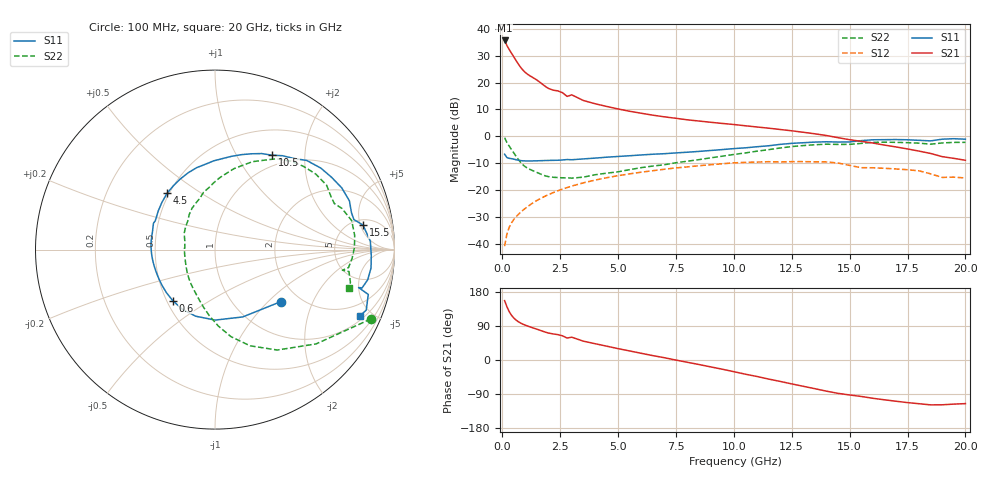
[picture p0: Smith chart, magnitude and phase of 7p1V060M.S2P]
! Infineon Technologies  Discrete & RF Semiconductors
! bfp620
! VCE =  1.0 V,  IC =  60 mA
! Common Emitter S-Parameters:  Sep 2002
# GHz  S  MA  R  50
!  f  S11  S21  S12  S22
! GHz  MAG  ANG  MAG  ANG  MAG  ANG  MAG  ANG
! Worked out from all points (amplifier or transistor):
!   59 points, 100 MHz to 20 GHz, reference 50 ohm
!   highest |S21| = 35.6 dB at 100 MHz (marker M1)
!   |S21| within 3 dB of that: start of sweep to 275 MHz
!   unconditionally stable (mu >= 1): 2.179 GHz to 2.203 GHz; 3.164 GHz to 10.1 GHz; 17.1 GHz to end of sweep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
!   at 1 GHz: K = 0.88, MSG = 25.2 dB, |S12| = -26.6 dB
!   at 5.5 GHz: K = 1.04, MAG = 10.4 dB, |S12| = -13.9 dB
!   at 20 GHz: K = 1.40, MAG = -0.5 dB, |S12| = -15.4 dB
!   S11 on the Smith chart (normalised r, x): 100 MHz: 1.62, -1.20; 600 MHz: 0.54, -0.35; 4.5 GHz: 0.49, +0.37; 10.5 GHz: 0.84, +1.42; 15.5 GHz: 6.10, +5.53; 20 GHz: 1.21, -4.26
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0.1  0.4679 -38.2  60.41 156.7  0.0092 79.1  0.9505 -24.0
0.2  0.4058 -67.6  48.66 140.4  0.0155 68.6  0.7704 -43.0
0.3  0.3927 -89.9  40.96 127.5  0.0207 64.9  0.6584 -58.2
0.4  0.3865 -106.2  34.94 117.8  0.0251 63.1  0.5703 -70.0
0.5  0.3784 -119.0  29.8 110.6  0.0289 62.1  0.493 -79.6
0.6  0.3693 -129.6  25.41 105.1  0.0325 61.6  0.4258 -87.6
0.7  0.3616 -138.5  21.8 100.7  0.036 61.4  0.3703 -94.8
0.8  0.3561 -145.9  18.97 97.2  0.0395 61.3  0.3271 -101.3
1  0.3511 -156.8  15.3 91.7  0.0466 61.1  0.2724 -112.2
1.4  0.3522 -170.6  11.82 83.2  0.0613 59.8  0.2238 -129.0
1.8  0.3567 177.4  8.851 74.8  0.076 57.4  0.1893 -147.6
2  0.3588 172.3  7.758 71.1  0.0833 56.0  0.1793 -156.2
2.8  0.373 156.8  5.527 57.9  0.1127 49.2  0.1705 177.1
3  0.3694 154.3  5.912 60.2  0.1199 47.3  0.1683 177.2
3.5  0.3828 145.6  4.648 49.7  0.1377 42.3  0.1756 163.5
4.5  0.4119 130.5  3.607 36.6  0.1711 32.3  0.2081 141.5
7  0.4786 96.4  2.311 6.0  0.2462 6.5  0.2985 106.3
10.5  0.6148 58.8  1.577 -37.5  0.3306 -33.9  0.4944 71.8
13.5  0.7854 26.0  1.119 -75.7  0.3382 -69.9  0.7015 36.9
15.5  0.8359 9.4  0.811 -96.2  0.263 -92.0  0.7432 18.0
17  0.8754 -6.7  0.639 -108.8  0.2492 -101.1  0.7769 0.8
20  0.8883 -24.6  0.361 -115.1  0.1699 -111.5  0.7763 -16.2
